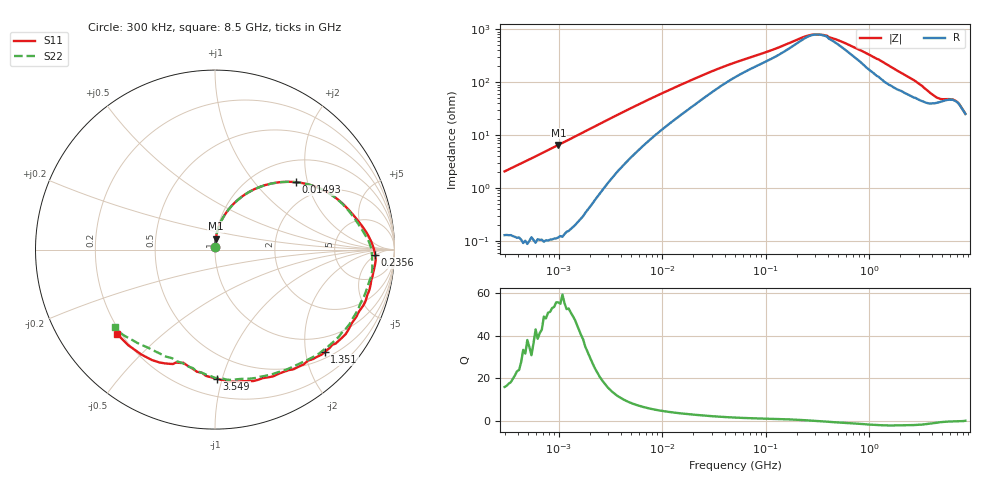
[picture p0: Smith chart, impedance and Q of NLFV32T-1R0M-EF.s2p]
! S-parameter Generated by TDK Corporation
! Copyright(C) 2015 TDK Corporation.
! All Rights Reserved.
! TDK P/N: NLFV32T-1R0M-EF (Inductors)
! Property: L=1uH at 7.96MHz
! Size(LxWxT): 3.2x2.5x2.2mm, 0.126x0.098x0.087inches
! Model Type: s2p (Touchstone File Format Version 1.0)
! Frequency: DC=Yes Start=0.3MHz Stop=8500MHz 225points Log-sweep
! Note:
! Model Generated on Jun. 23, 2015
! Hash(MD5):
! Port Assignments:
!  1 ---@@@--- 2
! Applicable Conditions:
!  Temperature = 25 degC
!  DC Bias Current = 0 A
!  Small Signal Operation
! Terms and conditions regarding TDK Simulation Models
! (1)This simulation model is being provided solely for informational purposes. Please refer to the specifications of the products in terms of detailed characteristics of such products.
! (2)In no event shall TDK Corporation of any of its subsidiaries be liable for any loss or damage arising, directly or indirectly,
!  From any information contained in this simulation model, including, but not limited to loss or damages arising from any inaccuracies, omissions or errors in connection with such information.
! (3)Any and all copyrights on this simulation model are owned by TDK Corporation.
!  Duplication or redistribution of this simulation model without prior written permission from TDK Corporation is prohibited.
! (4)This simulation model is subject to any modification or change without any prior notice.
! (5)Neither TDK Corporation nor any of its subsidiaries shall make any warranty, express or implied,
!  Including but not limited to the correctness, implied warranties of merchantability and fitness for a particular purpose with respect to this simulation models.
! (6)The use of this simulation model shall be deemed to have consented to the terms and conditions hereof.
# MHz S MA R 50
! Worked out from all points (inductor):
!   224 points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, 300 kHz to 8.5 GHz, reference 50 ohm
!   read as one part in series: L = 1.08 uH near 314.1 kHz
!   highest Q = 55.5 at 991.3 kHz (marker M1), where L = 1.04 uH
!   self-resonance near 318 MHz
!   S11 on the Smith chart (normalised r, x): 300 kHz: 1.00, +0.03; 14.93 MHz: 1.48, +1.70; 235.6 MHz: 16, -5; 1.351 GHz: 0.63, -2.40; 3.549 GHz: 0.32, -0.96; 8.5 GHz: 0.18, -0.36
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0.3  0.01629 86.8  0.9971 -1.2  0.9996 -1.7  0.01627 84.3
0.9913414  0.06184 85.7  0.996 -3.7  0.9979 -4.1  0.06168 85.3
1.72111  0.1091 82.3  0.9902 -6.3  0.9926 -6.7  0.109 82.1
4.316363  0.2616 69.1  0.939 -15.1  0.9408 -15.6  0.2616 69.0
9.430415  0.4651 51.2  0.7978 -27.3  0.7992 -27.7  0.4657 51.1
14.93432  0.5871 39.8  0.6684 -34.8  0.6693 -35.2  0.5879 39.7
28.42509  0.7178 25.1  0.4717 -42.0  0.4725 -42.4  0.7177 25.0
51.67171  0.7865 15.2  0.33 -42.6  0.3306 -43.0  0.7827 15.0
118.2037  0.8514 6.1  0.2056 -39.6  0.206 -40.0  0.8394 5.8
235.5662  0.8931 -1.9  0.123 -24.0  0.1232 -24.5  0.876 -2.3
283.1228  0.8967 -4.4  0.1126 -13.6  0.1128 -13.9  0.8797 -4.8
390.6008  0.8903 -9.5  0.1167 6.9  0.1171 6.5  0.8827 -9.8
647.669  0.8839 -20.3  0.1699 25.6  0.1703 25.3  0.8638 -20.7
979.5854  0.8669 -31.0  0.2366 28.5  0.236 27.5  0.8502 -31.8
1351.452  0.836 -42.9  0.3011 22.7  0.3018 22.2  0.8232 -42.9
1551.304  0.8181 -48.3  0.332 18.7  0.3326 17.6  0.8063 -48.7
2693.286  0.7625 -73.8  0.4261 -4.5  0.4257 -6.0  0.7449 -74.9
3548.748  0.7204 -89.1  0.4628 -19.8  0.4651 -20.6  0.7153 -89.9
4895.91  0.66 -104.5  0.4649 -43.7  0.4666 -44.9  0.6603 -104.7
6754.475  0.6924 -113.7  0.3873 -64.5  0.3882 -65.3  0.6635 -125.2
7753.325  0.7143 -125.1  0.3718 -69.6  0.3729 -72.6  0.6976 -136.7
8500  0.7203 -139.3  0.3661 -78.7  0.3656 -78.4  0.7045 -142.5
